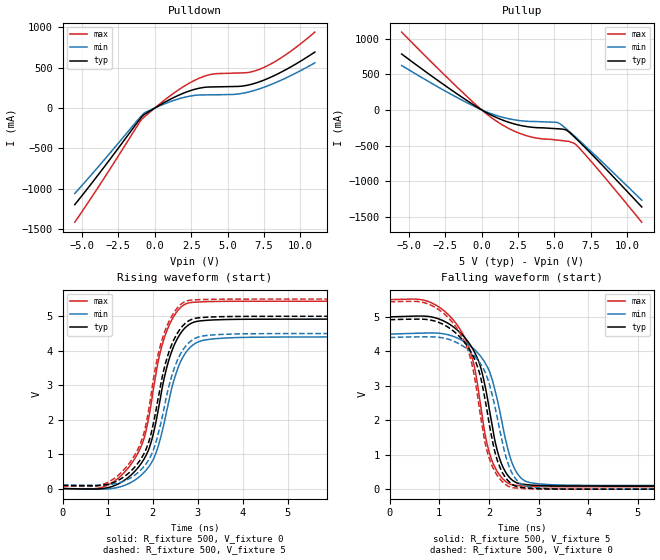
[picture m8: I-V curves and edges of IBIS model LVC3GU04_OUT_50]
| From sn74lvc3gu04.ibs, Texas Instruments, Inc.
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[Model]   LVC3GU04_OUT_50
Model_type  Output
Vref =   0
Rref =   500
Cref =   50p
Vmeas =   2.5
| variable   typ   min   max
C_comp   11.46pF   6.14pF   17.84pF
| C_pullup   13.27pF   6.14pF   17.84pF
| C_pulldown   9.64pF   6.21pF   13.79pF
[Temperature Range]   40   100   -40
| Ambient temperature   25   85   -40
[Voltage range]   5   4.5   5.5
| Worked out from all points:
|   slope of the pulldown table from 0 to 0.75 V, typ, clamps not added: 9.57 ohm
|   slope of the pullup table from 0 to 0.75 V, typ, clamps not added: 9.16 ohm
|   rising waveform, R_fixture 500, V_fixture 0: 20-80 % time 551ps typ, 543ps min, 557ps max; typ from 0 V to 4.92 V
|   falling waveform, R_fixture 500, V_fixture 5: 20-80 % time 483ps typ, 474ps min, 483ps max; typ from 5 V to 0.09 V
|   rising waveform, R_fixture 500, V_fixture 5: 20-80 % time 548ps typ, 545ps min, 554ps max; typ from 0.09 V to 5 V
|   falling waveform, R_fixture 500, V_fixture 0: 20-80 % time 483ps typ, 476ps min, 483ps max; typ from 4.92 V to 0 V
[Pulldown]
| LVC3GU04_OUT_50
|   Voltage   I(typ)   I(min)   I(max)
-5.5V     -1.198A    -1.059A    -1.415A
-945mV    -119.5mA   -101.1mA   -149.8mA
-655mV    -72.12mA   -54.5mA    -99.76mA
595mV     62.92mA    46.46mA    88.01mA
2.135V    195.6mA    137.1mA    283.5mA
3.44V     257mA      162.7mA    396.3mA
4.165V    262.1mA    164.5mA    425.2mA
5.735V    267.9mA    174.3mA    434.2mA
6.595V    292.3mA    205.6mA    446.8mA
7.495V    345.8mA    257.1mA    502.8mA
9.075V    482.4mA    378.2mA    670mA
11V       693.7mA    560.3mA    941.4mA
[Pullup]
| LVC3GU04_OUT_50
|   Voltage   I(typ)   I(min)   I(max)
-5.5V     783.3mA    622.7mA    1.091A
-1.19V    155.4mA    119.2mA    222.1mA
15mV      -1.802mA   -1.349mA   -2.612mA
915mV     -97.72mA   -71.78mA   -143.9mA
1.95V     -179.4mA   -128mA     -269.6mA
2.99V     -230.7mA   -157.8mA   -356.2mA
3.915V    -250.3mA   -165mA     -399.7mA
5.305V    -266mA     -186mA     -425.6mA
5.83V     -285.1mA   -268.2mA   -437.7mA
6.535V    -412.1mA   -396.1mA   -498.9mA
8.11V     -738.1mA   -697.5mA   -862.8mA
11V       -1.361A    -1.267A    -1.575A
[Ramp]
| LVC3GU04_OUT_50
| variable   typ   min   max
dV/dt_r   2.96/5.59E-10   2.65/5.48E-10   3.27/5.66E-10
dV/dt_f   2.96/4.96E-10   2.66/4.87E-10   3.27/4.92E-10
R_load = 500
[Rising Waveform]
| LVC3GU04_OUT_50
R_fixture =   500
C_fixture =   0
L_fixture =   0
V_fixture =   0
V_fixture_min = 0
V_fixture_max = 0
|   Time   V(typ)   V(min)   V(max)
0s        48.17pV    4.011nV    1.536nV
1.015ns   29.16mV    -7.084mV   108.8mV
1.705ns   660mV      345.2mV    1.117V
1.835ns   924.5mV    508.3mV    1.589V
1.97ns    1.377V     748.5mV    2.51V
2.265ns   3.264V     1.975V     4.406V
2.53ns    4.308V     3.39V      5.121V
2.815ns   4.768V     4.077V     5.392V
4.295ns   4.915V     4.393V     5.437V
24.99ns   4.917V     4.401V     5.437V
[Falling Waveform]
| LVC3GU04_OUT_50
R_fixture =   500
C_fixture =   0
L_fixture =   0
V_fixture =   5
V_fixture_min = 4.5
V_fixture_max = 5.5
|   Time   V(typ)   V(min)   V(max)
0s        5V         4.5V       5.5V
920ps     4.973V     4.532V     5.351V
1.565ns   4.306V     4.221V     4.23V
1.82ns    3.6V       3.878V     2.556V
2.035ns   2.097V     3.318V     936.2mV
2.235ns   806mV      2.147V     373.4mV
2.495ns   236.4mV    661.5mV    117.8mV
2.775ns   129.1mV    208.8mV    85.65mV
3.575ns   91.6mV     115.4mV    71.74mV
24.99ns   89.62mV    107.6mV    71.33mV
[Rising Waveform]
| LVC3GU04_OUT_50
R_fixture =   500
C_fixture =   0
L_fixture =   0
V_fixture =   5
V_fixture_min = 4.5
V_fixture_max = 5.5
|   Time   V(typ)   V(min)   V(max)
0s        89.62mV    107.6mV    71.33mV
995ps     122.8mV    109.9mV    175.6mV
1.665ns   727.8mV    456mV      1.131V
1.935ns   1.456V     888.8mV    2.488V
2.1ns     2.477V     1.482V     3.773V
2.25ns    3.467V     2.319V     4.499V
2.505ns   4.411V     3.587V     5.173V
2.805ns   4.873V     4.236V     5.461V
4.22ns    4.998V     4.494V     5.5V
24.99ns   5V         4.5V       5.5V
[Falling Waveform]
| LVC3GU04_OUT_50
R_fixture =   500
C_fixture =   0
L_fixture =   0
V_fixture =   0
V_fixture_min = 0
V_fixture_max = 0
|   Time   V(typ)   V(min)   V(max)
0s        4.917V     4.401V     5.437V
895ps     4.884V     4.418V     5.294V
1.525ns   4.23V      4.103V     4.22V
1.67ns    3.894V     3.923V     3.542V
1.81ns    3.368V     3.682V     2.31V
1.995ns   1.988V     3.109V     943.5mV
2.19ns    748.7mV    1.918V     352.5mV
2.485ns   125.4mV    414mV      41.11mV
3.57ns    1.543mV    5.659mV    339.7uV
24.99ns   2.295nV    8.463nV    2.471nV
